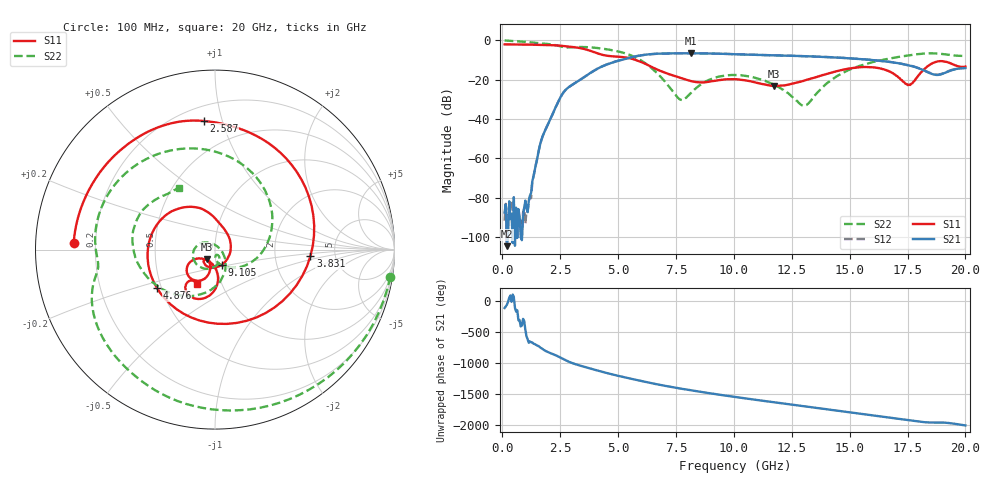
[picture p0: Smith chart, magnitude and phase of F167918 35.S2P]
!  2-Port S-parameters saved by WinCal
! VAR MeasName=S-Parameters (CALIBRATED_DATA) read from VNA (N5242A)
! VAR MeasDate=2016-11-22 10:26:26
! VAR NAME=F167918 35
! VAR FILENAME=F167918 35.S2P
! VAR DATE=2016-11-22 10:26:26
! VAR PHYS_PORTS=1,2
# Hz S DB R 50
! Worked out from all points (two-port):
!   401 points, 100 MHz to 20 GHz, reference 50 ohm
!   highest |S21| = -6.61 dB at 8.159 GHz (marker M1); lowest = -104.5 dB at 199.5 MHz (marker M2)
!   |S21| within 3 dB of the highest: 5.247 GHz to 15.5 GHz (10.26 GHz wide, 98.9 % of centre)
!   lowest |S11| = -23.2 dB at 11.74 GHz (marker M3), VSWR 1.15, Z = 45.6 - j4.96 ohm
!   |S11| at or under -10 dB: 5.76 GHz to end of sweep
!   |S22| runs from -33.3 to -0.1 dB; largest |S21 - S12| = 0.0041
!   S11 on the Smith chart (normalised r, x): 100 MHz: 0.12, +0.02; 2.587 GHz: 0.29, +0.87; 3.831 GHz: 3.24, -0.33; 4.876 GHz: 0.47, -0.24; 9.105 GHz: 1.06, -0.18; 20 GHz: 0.76, -0.30
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1e8  -2.07 177.3  -87.38 -113.2  -91.59 33.6  -0.10 -8.8
1.995e8  -2.08 174.6  -104.50 -60.6  -102.53 8.3  -0.16 -17.0
1.14475e9  -2.23 149.0  -81.43 45.3  -81.68 55.4  -0.96 -87.8
1.74175e9  -2.35 130.4  -48.74 -57.3  -48.74 -56.8  -1.63 -124.6
2.5875e9  -2.86 95.1  -27.42 151.8  -27.43 151.6  -3.37 -167.9
3.43325e9  -4.15 39.0  -19.50 28.5  -19.52 28.6  -3.41 161.1
3.83125e9  -5.47 -4.0  -16.37 -13.5  -16.37 -13.3  -3.62 142.2
4.32875e9  -7.41 -73.6  -13.20 -65.1  -13.14 -65.0  -4.26 117.4
4.876e9  -8.23 -146.7  -10.86 -117.3  -10.81 -117.5  -5.35 87.8
5.82125e9  -10.26 132.2  -7.99 162.4  -8.01 162.0  -9.13 24.4
6.7665e9  -15.22 89.4  -6.78 88.4  -6.82 88.3  -17.66 -51.2
7.662e9  -19.00 52.9  -6.62 27.9  -6.65 28.0  -29.98 -80.3
8.1595e9  -20.76 17.2  -6.61 -2.8  -6.63 -2.9  -26.63 -59.8
9.10475e9  -20.72 -65.2  -6.75 -58.1  -6.74 -58.2  -19.29 -103.7
1.005e10  -19.77 -116.7  -7.07 -109.9  -7.07 -109.9  -17.63 -150.0
1.17415e10  -23.18 -128.7  -7.66 164.3  -7.64 164.2  -22.48 148.3
1.338325e10  -19.31 -103.9  -8.21 83.1  -8.18 83.2  -29.75 -3.5
1.497525e10  -14.34 -116.0  -9.17 4.6  -9.12 4.3  -15.06 -80.1
1.67165e10  -15.86 -152.6  -10.93 -82.9  -11.00 -83.0  -9.28 -135.0
1.756225e10  -22.57 -119.3  -12.73 -126.2  -12.66 -126.1  -7.63 -161.2
1.87065e10  -11.04 -103.9  -17.55 -163.3  -17.43 -163.3  -6.67 156.7
2e10  -13.35 -118.3  -14.12 150.0  -14.00 149.8  -7.98 120.3
